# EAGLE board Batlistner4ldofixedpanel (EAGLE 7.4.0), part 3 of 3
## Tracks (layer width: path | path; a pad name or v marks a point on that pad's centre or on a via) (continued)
N$349  (via drill 0.5)  (1 unrouted) (continued)
  Top 0.406: IC34.19 v159.7,97.16 | v153.99,109.86 153.99,110.17 154.62,110.81 154.62,112.08
  Bottom 0.406: SCK5.TP 160.02,97.16 v159.7,97.16 157.8,97.16 153.99,100.97 v153.99,109.86
N$350  (via drill 0.5)  (1 unrouted)
  Top 0.406: R213.1 v155.89,109.85 | v160.66,100.65 160.97,100.33 IC34.18
  Bottom 0.406: MISO5.TP 164.47,97.16 162.56,99.06 160.66,99.06 | 160.66,99.06 157.48,99.06 154.94,101.6 154.94,109.86 v155.89,109.86 | 160.66,99.06 v160.66,100.65
N$351  (via drill 0.5)
  Top 0.406: R214.1 154.62,98.43 154.62,96.84 156.21,95.25 161.61,95.25 162.24,95.89 IC34.17 v162.24,100.33 | v167,96.52 167,92.08 166.05,91.12 v163.19,91.12
  Bottom 0.406: v162.24,100.33 163.19,100.33 v167,96.52 | v163.19,91.12 162.88,91.12 161.93,92.08 MOSI5.TP
N$352
  Top 0.406: R215.1 153.16,97.03 155.57,94.61 162.56,94.61 163.51,95.57 IC34.16
N$353
  Top 0.406: R216.1 162.24,102.23 164.78,99.69 IC34.15
N$354
  Top 0.406: IC34.14 166.05,100.01 161.73,104.33 R217.1
N$355  (via drill 0.5)
  Top 0.406: R218.1 v157.16,104.78 | v167.32,100.65 IC34.13
  Bottom 0.406: v157.16,104.78 161.29,104.78 163.19,102.87 165.1,102.87 v167.32,100.65
N$356  (1 unrouted)
  Top 0.406: IC34.12 168.59,101.92 168.28,102.23 168.12,102.39 167.64,102.87
N$357
  Top 0.406: R212.2 152.72,111.76 IC35.5
N$358
  Top 0.406: IC35.4 153.04,107.31 R213.2
N$359
  Top 0.406: IC35.10 146.69,99.69 147.96,100.97 152.72,100.97 R214.2
N$360
  Top 0.406: IC35.1 150.81,97.35 R215.2
N$361
  Top 0.406: IC35.2 R216.2
N$362
  Top 0.406: IC35.3 151.45,104.78 152.72,106.05 157.99,106.05 R217.2
N$363
  Top 0.406: IC35.8 144.46,104.78 145.73,103.5 152.4,103.5 R218.2
N$364
  Top 0.406: IC35.7 145.1,107.31 146.37,106.05 151.76,106.05 152.4,106.68 158.43,106.68 159.23,105.89 162.72,105.89 162.88,105.73 162.88,104.62 164.94,102.55 R219.2
N$365  (via drill 0.5)
  Top 0.406: v165.42,87.95 R233.2
  Bottom 0.406: IC35.9 144.46,102.23 145.41,101.28 145.41,98.42 147.32,96.52 147.32,95.25 149.22,93.34 149.22,90.81 152.08,87.95 v165.42,87.95
N$366  (via drill 0.5)
  Top 0.406: R234.2 157.64,86.2 155.57,88.27 153.03,88.27 v151.76,89.53
  Bottom 0.406: v151.76,89.53 151.76,94.61 146.05,100.33 146.05,108.58 144.78,109.86 IC35.6
N$367
  Top 0.406: C238.1 149.91,92.03 150.5,91.44 151.42,91.44 X6.3 151.49,91.08 153.35,89.22 155.89,89.22 157.48,87.63 162.56,87.63 163.51,88.58 IC34.5
N$368  (via drill 0.5)
  Top 0.406: IC34.20 158.43,100.01 158.75,100.33 v158.75,100.65 C239.2 | v175.26,102.23 176.53,102.23 176.65,102.12 | R224.1 172.09,92.71 v168.91,95.89 | R220.1 177.8,100.97 176.65,102.12 | C240.1 178.44,102.87 | 178.44,102.87 177.4,102.87 176.65,102.12 | 176.65,102.12 | IC36.3 178.44,104.54 178.44,102.87
  Bottom 0.406: v175.26,102.23 170.81,102.23 168.91,100.33 168.91,98.42 | VCC5.TP 165.74,92.71 v168.91,95.89 168.91,98.42 | 168.91,98.42 167.64,98.42 163.83,102.23 158.75,102.23 v158.75,100.65
N$369
  Top 0.406: R222.1 184.78,97.16 183.51,98.42 181.5,98.42 C242.1 177.98,98.57 R220.2 177.48,98.42 R221.1
N$370
  Top 0.406: C243.2 179.71,90.66 Q23.B R222.2
N$371
  Top 0.406: Q23.C 176.8,93.34 C244.1 176.53,94.61 175.58,95.57 R221.2
N$372
  Top 0.406: C266.1 C241.1 180.97,107.05 | 180.97,107.05 177.01,107.05 IC36.2@1 | R223.2 180.97,109.22 180.97,107.05
N$373  (via drill 0.5)
  Top 0.406: IC34.1 158.17,89.48 v156.21,91.44
  Bottom 0.406: v156.21,91.44 156.21,93.98 157.48,95.25 RES5.TP
N$374
  Top 0.406: IC34.9 168.59,87.95 168.91,87.63 171.13,87.63 171.77,88.27 171.77,91.12 R224.2 173.04,91.44 173.99,91.44 173.68,91.12 R225.1 174.04,91.08 C244.2
N$375
  Top 0.406: R226.1 176.85,68.9 C245.2
N$376
  Top 0.406: IC33.1 175.52,74.87 | 175.52,74.87 R226.2 | 175.52,74.87 175.52,75.51 C268.1
N$377
  Top 0.406: R227.2 179.38,86.94 C243.1
N$378  (via drill 0.5)
  Top 0.406: C250.2 R228.1 184.47,86.36 181.29,83.19 v177.8,83.19 | 163.83,80.64 161.29,80.64 159.38,78.74 R205.1 v159.38,81.28 | 163.83,80.64 166.69,80.64 168.28,82.07 168.28,82.55 168.91,83.19 v171.45,83.19 172.09,82.55 R200.1 | IC32.7 163.83,80.64 | IC31.8 149.86,83.82 150.5,83.19 v151.13,83.19
  Bottom 0.406: v171.45,83.19 173.35,85.09 175.9,85.09 v177.8,83.19 | v151.13,83.19 151.76,83.19 152.4,82.55 158.12,82.55 v159.38,81.28
N$379
  Top 0.406: R223.1 R229.2 187.01,108.9 187.96,107.95 C251.1
N$380
  Top 0.406: SG12.+ 146.37,73.66 147,73.03 C267.2
N$381
  Top 0.406: R230.1 C267.1 150.03,71.12 Q24.B
N$382
  Top 0.406: C268.2 R231.1
N$383
  Top 0.406: R231.2 175.57,77.78 177.16,79.38 IC33.8
N$384
  Top 0.406: U$6.P$1 196.53,65.22 R232.2
N$385
  Top 0.406: U$6.P$5 187.17,72.24 187.48,72.55 190.34,72.56 191.13,71.75 193.65,71.75 U$6.P$6 194.61,72.06 SP6.+
N$386
  Top 0.406: C237.1 153.03,94.61 153.03,92.71 | 153.03,92.71 153.03,90.81 153.67,90.17 155.89,90.17 157.8,88.27 161.93,88.27 162.24,88.58 IC34.4 | X6.1 153.1,92.78 153.03,92.71
N$387
  Top 0.406: IC34.6 164.78,88.58 163.04,86.84 163.04,86.52 R234.1
N$388
  Top 0.406: R233.1 167.32,87.47 166.05,88.74 IC34.7
N$389
  Top 0.406: S6.3 186.55,111.9 187.32,111.12 190.5,111.12 191.77,109.86 D6.A 192.65,108.58 C270.1 C269.1
N$390
  Top 0.406: S6.2 189.69,113.84 192.41,111.12 194.31,111.12 194.94,110.49 197.49,110.49 198.12,109.86 198.12,104.14 G6.+

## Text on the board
Bottom: BAT- | BAT- | BAT- | LISTENER IV + | LISTENER IV + | LISTENER IV + | BAT- | BAT- | BAT- | LISTENER IV + | LISTENER IV + | LISTENER IV +
tPlace: - | - | - | - | - | -
tNames: o | o | o | o | o | o | o | o | o | o | + | o | + | o | + | o | o | o | o | o | o | o | o | o | o | + | o | + | o | +
bNames: AND LED DISPLAY BY PE1PWF | AND LED DISPLAY BY PE1PWF | AND LED DISPLAY BY PE1PWF | BAT DETECTOR 25+40KHZ UST | - | BAT DETECTOR 25+40KHZ UST | - | BAT DETECTOR 25+40KHZ UST | - | AND LED DISPLAY BY PE1PWF | AND LED DISPLAY BY PE1PWF | AND LED DISPLAY BY PE1PWF | BAT DETECTOR 25+40KHZ UST | - | BAT DETECTOR 25+40KHZ UST | - | BAT DETECTOR 25+40KHZ UST | -
_tPlace: R18 | R18 | R18 | R17 | R17 | R17 | R18 | R18 | R18 | R17 | R17 | R17
_tNames: R15 | R15 | R15 | S1 | S1 | S1 | C19 | R30 | C41 | R35 | C19 | R30 | C41 | R35 | C19 | R30 | C41 | R35 | R19 | R19 | R19 | D1 | D1 | D1 | R23 | C28 | C45 | R23 | C28 | C45 | R23 | C28 | C45 | IC6 | C44 | IC6 | C44 | IC6 | C44 | R24 | R24 | R24 | C18 | C1 | C29 | C18 | C1 | C29 | C18 | C1 | C29 | C17 | R26 | C17 | R26 | C17 | R26 | R22 | R27 | R22 | R27 | R22 | R27 | IC5 | R20 | R25 | IC5 | R20 | R25 | IC5 | R20 | R25 | C31 | C30 | C31 | C30 | C31 | C30 | C20 | C20 | C20 | R21 | R29 | R21 | R29 | R21 | R29 | C4 | Q4 | R28 | C4 | Q4 | R28 | C4 | Q4 | R28 | R31 | R31 | R31 | IC4 | C22 | G1 | IC4 | C22 | G1 | IC4 | C22 | G1 | X1 | X1 | X1 | C11 | C27 | C11 | C27 | C11 | C27 | C16 | IC1 | C16 | IC1 | C16 | IC1 | R34 | R34 | R34 | R9 | R9 | R9 | C21 | C21 | C21 | R40 | R39 | C10 | R40 | R39 | C10 | R40 | R39 | C10 | IC2 | R12 | R33 | IC3 | IC2 | R12 | R33 | IC3 | IC2 | R12 | R33 | IC3 | C9 | C9 | C9 | C5 | C5 | C5 | R8 | C15 | R8 | C15 | R8 | C15 | R3 | C12 | R11 | R3 | C12 | R11 | R3 | C12 | R11 | R1 | C8 | R13 | R1 | C8 | R13 | R1 | C8 | R13 | R2 | R10 | R2 | R10 | R2 | R10 | C43 | C43 | C43 | R37 | C32 | R37 | C32 | R37 | C32 | Q2 | C3 | C40 | Q2 | C3 | C40 | Q2 | C3 | C40 | R4 | R4 | R4 | C6 | SP1 | C6 | SP1 | C6 | SP1 | C42 | Q3 | C25 | C2 | C13 | C14 | C42 | Q3 | C25 | C2 | C13 | C14 | C42 | Q3 | C25 | C2 | C13 | C14 | C26 | R32 | R38 | C26 | R32 | R38 | C26 | R32 | R38 | C24 | C24 | C24 | R7 | C23 | R7 | C23 | R7 | C23 | SG2 | Q1 | SG2 | Q1 | SG2 | Q1 | R36 | R6 | R36 | R6 | R36 | R6 | R5 | C7 | R5 | C7 | R5 | C7 | R14 | R14 | R14 | R15 | R15 | R15 | S1 | S1 | S1 | R19 | C19 | R30 | C41 | R35 | R19 | C19 | R30 | C41 | R35 | R19 | C19 | R30 | C41 | R35 | D1 | D1 | D1 | C45 | C45 | C45 | R23 | C28 | R23 | C28 | R23 | C28 | IC6 | C44 | IC6 | C44 | IC6 | C44 | R24 | R24 | R24 | C18 | C1 | C29 | C18 | C1 | C29 | C18 | C1 | C29 | C17 | R26 | C17 | R26 | C17 | R26 | R22 | R27 | R22 | R27 | R22 | R27 | IC5 | R20 | R25 | IC5 | R20 | R25 | IC5 | R20 | R25 | C31 | C30 | C31 | C30 | C31 | C30 | R29 | C20 | R29 | C20 | R29 | C20 | R21 | R21 | R21 | C4 | Q4 | R28 | C4 | Q4 | R28 | C4 | Q4 | R28 | R31 | R31 | R31 | IC4 | C22 | G1 | IC4 | C22 | G1 | IC4 | C22 | G1 | X1 | X1 | X1 | C11 | C27 | C11 | C27 | C11 | C27 | C16 | IC1 | C16 | IC1 | C16 | IC1 | R34 | R34 | R34 | R9 | R9 | R9 | C10 | C21 | C10 | C21 | C10 | C21 | R40 | R39 | R40 | R39 | R40 | R39 | IC2 | R12 | R33 | IC3 | IC2 | R12 | R33 | IC3 | IC2 | R12 | R33 | IC3 | C9 | C9 | C9 | C5 | C5 | C5 | R8 | C15 | R8 | C15 | R8 | C15 | R3 | C12 | R11 | R3 | C12 | R11 | R3 | C12 | R11 | R1 | C8 | R13 | R1 | C8 | R13 | R1 | C8 | R13 | R2 | R10 | R2 | R10 | R2 | R10 | C43 | C43 | C43 | R37 | C32 | R37 | C32 | R37 | C32 | Q2 | C3 | C40 | Q2 | C3 | C40 | Q2 | C3 | C40 | R4 | R4 | R4 | C6 | C25 | C2 | SP1 | C6 | C25 | C2 | SP1 | C6 | C25 | C2 | SP1 | C42 | Q3 | C13 | C14 | C42 | Q3 | C13 | C14 | C42 | Q3 | C13 | C14 | C26 | R32 | R38 | C26 | R32 | R38 | C26 | R32 | R38 | C24 | C24 | C24 | R7 | C23 | R7 | C23 | R7 | C23 | SG2 | Q1 | SG2 | Q1 | SG2 | Q1 | R36 | R6 | R36 | R6 | R36 | R6 | R5 | C7 | R5 | C7 | R5 | C7 | R14 | R14 | R14
_bNames: RES | MISO | RES | MISO | RES | MISO | SCK | SCK | SCK | SG1 | GND | MOSI | VCC | SG1 | GND | MOSI | VCC | SG1 | GND | MOSI | VCC | RES | MISO | RES | MISO | RES | MISO | SCK | SCK | SCK | GND | GND | GND | SG1 | MOSI | VCC | SG1 | MOSI | VCC | SG1 | MOSI | VCC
